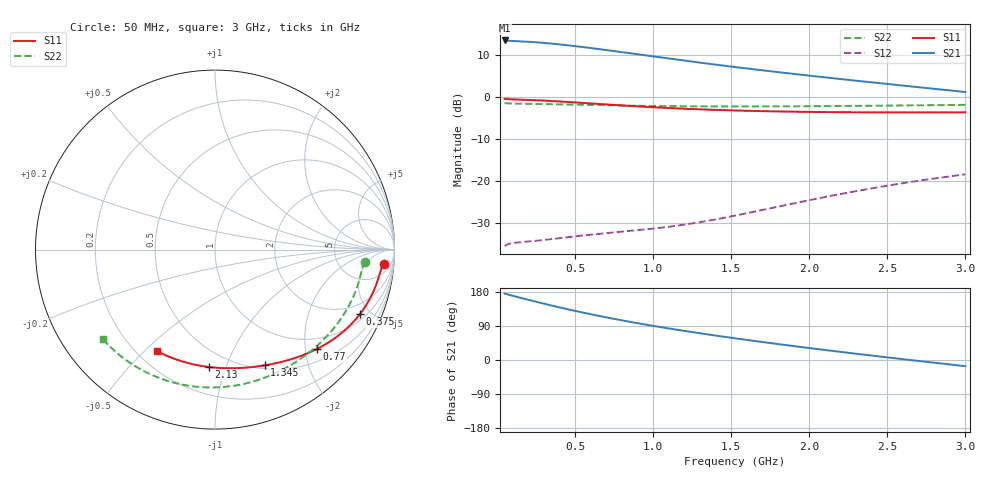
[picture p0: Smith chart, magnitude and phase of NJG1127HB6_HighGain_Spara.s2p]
! Created Mon Dec 09 19:53:09 2013
# hz S ma R 50
! 2 Port Network Data from SP1.SP block
! freq  magS11  angS11  magS21  angS21  magS12  angS12  magS22  angS22
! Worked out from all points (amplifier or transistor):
!   591 points, 50 MHz to 3 GHz, reference 50 ohm
!   highest |S21| = 13.4 dB at 50 MHz (marker M1)
!   |S21| within 3 dB of that: start of sweep to 842.9 MHz
!   unconditionally stable (mu >= 1): 96.59 MHz to 2.212 GHz
!   at 540 MHz: K = 1.18, MAG = 19.9 dB, |S12| = -33.1 dB
!   at 1.525 GHz: K = 1.41, MAG = 13.9 dB, |S12| = -28.3 dB
!   at 3 GHz: K = 0.71, MSG = 9.8 dB, |S12| = -18.5 dB
!   S11 on the Smith chart (normalised r, x): 50 MHz: 11, -16; 375 MHz: 1.31, -4.31; 770 MHz: 0.75, -2.25; 1.345 GHz: 0.54, -1.37; 2.13 GHz: 0.38, -0.88; 3 GHz: 0.28, -0.54
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5e7  0.9425 -5.0  4.672 175.5  0.01662 29.7  0.8389 -4.7
1.4e8  0.924 -10.0  4.577 165.3  0.01844 18.2  0.8257 -8.4
2.2e8  0.9128 -14.8  4.487 156.9  0.019 19.1  0.8216 -12.4
3e8  0.8989 -19.7  4.371 148.7  0.01967 21.5  0.8171 -16.5
3.75e8  0.8836 -24.1  4.244 141.4  0.02041 23.9  0.8123 -20.3
4.6e8  0.8645 -28.8  4.083 133.3  0.02131 26.5  0.8064 -24.5
5.45e8  0.8446 -33.4  3.912 125.6  0.0222 28.8  0.8003 -28.7
6.5e8  0.82 -38.6  3.695 116.6  0.02325 31.5  0.7931 -33.8
7.7e8  0.7932 -44.2  3.451 107.0  0.0244 34.7  0.7857 -39.4
9e8  0.7669 -49.9  3.199 97.2  0.0257 38.4  0.7789 -45.5
1.035e9  0.7431 -55.3  2.957 87.7  0.02732 42.6  0.7734 -51.6
1.185e9  0.7209 -61.0  2.713 77.7  0.02969 47.3  0.7691 -58.4
1.345e9  0.7017 -66.8  2.482 67.8  0.03315 52.0  0.7664 -65.6
1.525e9  0.685 -73.1  2.254 57.2  0.03837 56.0  0.7653 -73.7
1.64e9  0.6766 -76.9  2.124 50.7  0.04245 57.7  0.7656 -78.9
1.76e9  0.6694 -80.9  2 44.2  0.04729 58.8  0.7665 -84.4
2.02e9  0.6583 -89.3  1.764 30.5  0.05962 58.5  0.7705 -96.2
2.13e9  0.6551 -92.9  1.676 25.0  0.06547 57.6  0.7728 -101.3
2.32e9  0.6514 -98.9  1.536 15.6  0.0763 55.0  0.7776 -110.0
2.51e9  0.6495 -104.8  1.411 6.4  0.08783 51.4  0.7832 -118.8
2.755e9  0.6494 -112.4  1.266 -5.1  0.1033 45.5  0.7911 -130.1
3e9  0.6517 -119.9  1.136 -16.3  0.1191 38.7  0.7994 -141.5
